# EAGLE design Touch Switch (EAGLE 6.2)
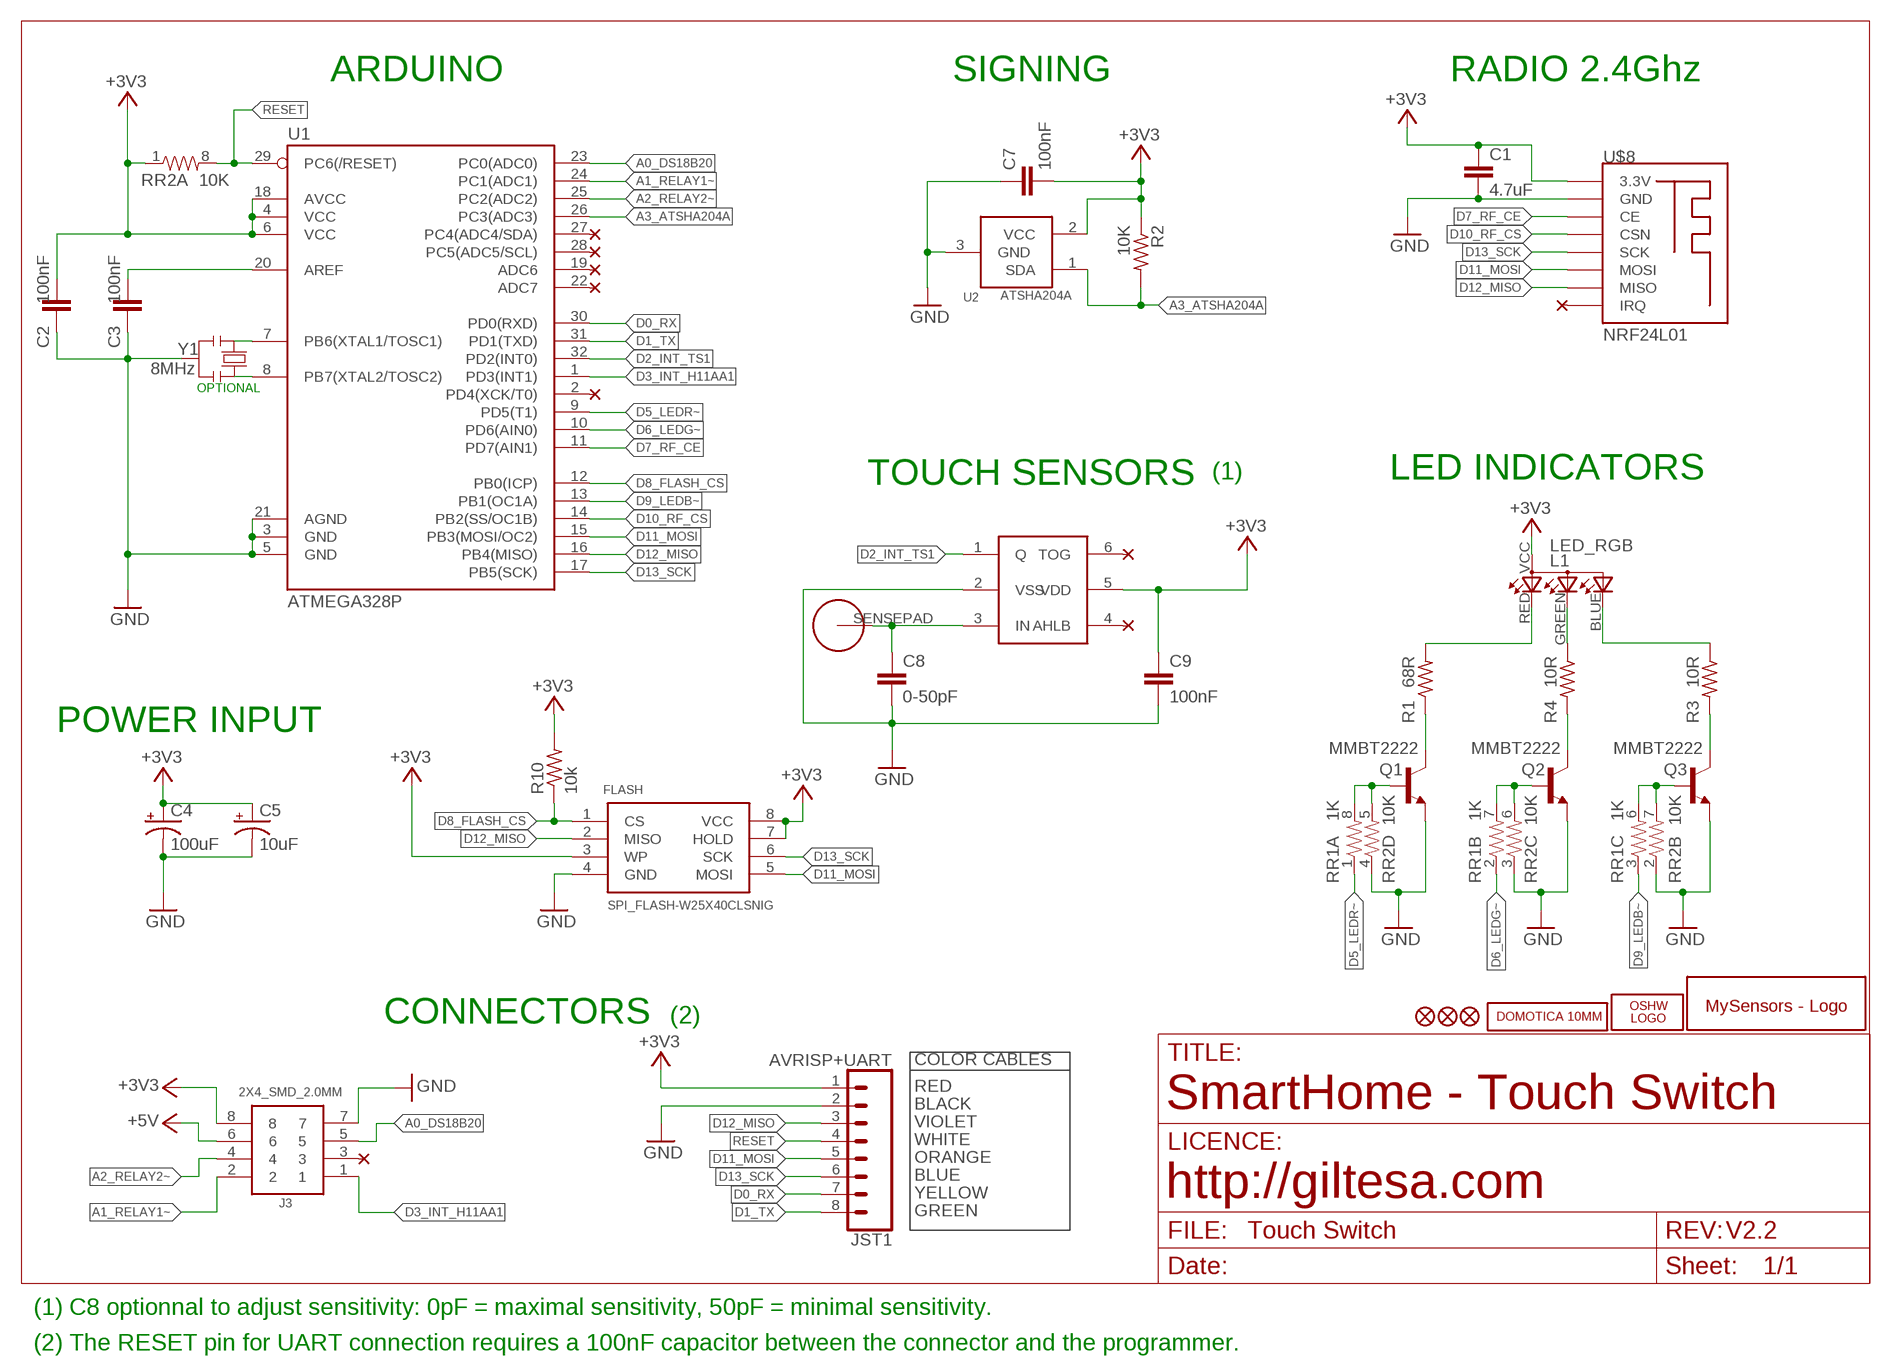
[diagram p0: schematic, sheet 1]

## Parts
C1  4.7uF  C1206  [C1206]
C2  100nF  C0603  [C0603]
C3  100nF  C0603  [C0603]
C4  100uF  10UF-16V-10%(TANT)  [EIA3216]
C5  10uF  10UF-16V-10%(TANT)  [EIA3216]
C7  100nF  C0603  [C0603]
C8  0-50pF  C0603  [C0603]
C9  100nF  C0603  [C0603]
FLASH  SPI_FLASH-W25X40CLSNIG  SPI_FLASH-X25XXSMD  [SO08]
J3  2X4_SMD_2.0MM  [2X4_SMD_2.0MM]
JST1  AVRISP+UART  JST-8-1MM-SMD  [JST-8-1MM-SMD]
L1  LED_RGB  LED_RGB_1206_SIDE  [LED_RGB_1206_SIDE]
LOGO1  OSHW_LOGO_FILLX0150-NT  [OSHW_FILLX150_NOTEXT]
Q1  MMBT2222  TRANSISTOR_NPNSOT23  [SOT23]
Q2  MMBT2222  TRANSISTOR_NPNSOT23  [SOT23]
Q3  MMBT2222  TRANSISTOR_NPNSOT23  [SOT23]
R1  68R  R0603  [R0603]
R2  10K  R0603  [R0603]
R3  10R  R0603  [R0603]
R4  10R  R0603  [R0603]
R10  10k  R0603  [R0603]
RR1  1K  RESISTOR-ARRAY0603-ARV  [0603-ARV]
RR2  10K  RESISTOR-ARRAY0603-ARV  [0603-ARV]
TTP1  TTP223  TTP223-BA6  [SOT-23-6]
U1  ATMEGA328P  ATMEGA328P_TQFP  [TQFP32-08]
U2  ATSHA204A  IC_ATSHA204A_CRYPT  [SOT23-3]
U$1  HTTM_SENSEPAD  [HTTM_SENSEPAD]
U$2  MYSENSORS  [MYSENSORS]
U$5  DOMOTICA-10MM  [DOMOTICA-10MM]
U$6  FIDUCIAL1X2  [FIDUCIAL-1X2]
U$7  FIDUCIAL1X2  [FIDUCIAL-1X2]
U$8  NRF24L01  NRF24L01_SMD  [NRF24L01_SMD]
U$14  FIDUCIAL1X2  [FIDUCIAL-1X2]
Y1  8MHz  RESONATORMU  [RESONATOR]

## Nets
+3V3: C1.1 C2.2 C4.A(+) C5.A(+) C7.2 C9.1 FLASH.3(WP) FLASH.7(HOLD) FLASH.8(VCC) J3.8 JST1.1 L1.VCC R2.1 R10.2 RR2.1 TTP1.5(VDD) U1.4(VCC) U1.6(VCC) U1.18(AVCC) U2.2(VCC) U$8.3.3V
+5V: J3.6
A0_DS18B20: J3.5 U1.23(PC0(ADC0))
A1_RELAY1~: J3.2 U1.24(PC1(ADC1))
A2_RELAY2~: J3.4 U1.25(PC2(ADC2))
A3_ATSHA204A: R2.2 U1.26(PC3(ADC3)) U2.1(SDA)
D0_RX: JST1.7 U1.30(PD0(RXD))
D1_TX: JST1.8 U1.31(PD1(TXD))
D2_INT_TS1: TTP1.1(Q) U1.32(PD2(INT0))
D3_INT_H11AA1: J3.1 U1.1(PD3(INT1))
D5_LEDR~: RR1.1 U1.9(PD5(T1))
D6_LEDG~: RR1.2 U1.10(PD6(AIN0))
D7_RF_CE: U1.11(PD7(AIN1)) U$8.CE
D8_FLASH_CS: FLASH.1(CS) R10.1 U1.12(PB0(ICP))
D9_LEDB~: RR1.3 U1.13(PB1(OC1A))
D10_RF_CS: U1.14(PB2(SS/OC1B)) U$8.CSN
D11_MOSI: FLASH.5(MOSI) JST1.5 U1.15(PB3(MOSI/OC2)) U$8.MOSI
D12_MISO: FLASH.2(MISO) JST1.3 U1.16(PB4(MISO)) U$8.MISO
D13_SCK: FLASH.6(SCK) JST1.6 U1.17(PB5(SCK)) U$8.SCK
GND: C1.2 C2.1 C3.1 C4.C(-) C5.C(-) C7.1 C8.2 C9.2 FLASH.4(GND) J3.7 JST1.2 Q1.2(E) Q2.2(E) Q3.2(E) RR2.2 RR2.3 RR2.4 TTP1.2(VSS) U1.3(GND) U1.5(GND) U1.21(AGND) U2.3(GND) U$8.GND Y1.2
N$1: Q1.3(C) R1.1
N$2: L1.GREEN R4.1
N$4: L1.RED R1.2
N$5: Q2.1(B) RR1.7 RR2.6
N$6: Q1.1(B) RR1.8 RR2.5
N$7: Q2.3(C) R4.2
N$8: Q3.3(C) R3.2
N$9: Q3.1(B) RR1.6 RR2.7
N$10: C8.1 TTP1.3(IN) U$1.SENSEPAD
N$11: L1.BLUE R3.1
N$29: U1.7(PB6(XTAL1/TOSC1)) Y1.1
N$30: U1.8(PB7(XTAL2/TOSC2)) Y1.3
N$33: C3.2 U1.20(AREF)
RESET: JST1.4 RR2.8 U1.29(PC6(/RESET))
Unconnected: J3.3 RR1.4 RR1.5 TTP1.4(AHLB) TTP1.6(TOG) U1.2(PD4(XCK/T0)) U1.19(ADC6) U1.22(ADC7) U1.27(PC4(ADC4/SDA)) U1.28(PC5(ADC5/SCL)) U$8.IRQ

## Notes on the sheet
- ARDUINO | SIGNING | RADIO 2.4Ghz
- OPTIONAL
- TOUCH SENSORS | (1) | LED INDICATORS
- POWER INPUT
- CONNECTORS | (2)
- COLOR CABLES
- RED
- BLACK | SmartHome - Touch Switch
- VIOLET
- WHITE
- ORANGE
- BLUE
- YELLOW | http://giltesa.com
- GREEN
- V2.2
- (1) C8 optionnal to adjust sensitivity: 0pF = maximal sensitivity, 50pF = minimal sensitivity.
- (2) The RESET pin for UART connection requires a 100nF capacitor between the connector and the programmer.

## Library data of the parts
C1 = ,giltesa:C1206
C2 C3 C7-C9 = ,giltesa:C0603
C4 = SparkFun-Capacitors:10UF-16V-10%(TANT): CAP-00811; PROD_ID: CAP-00811; VALUE: 10uF
C5 = SparkFun-Capacitors:10UF-16V-10%(TANT): CAP-00811; PROD_ID: CAP-00811
FLASH = SparkFun-DigitalIC:SPI_FLASH-X25XX: 8pin SPI Flash series x25xx. Works with devices like W25X32 and BR25L32
J3 = ,giltesa:2X4_SMD_2.0MM
JST1 = ,giltesa:JST-8-1MM-SMD
L1 = ,giltesa:LED_RGB_1206_SIDE
LOGO1 = ohw-logo:OSHW_LOGO_FILL
Q1-Q3 = SparkFun:TRANSISTOR_NPN: Transistor NPN BJT configuration in SOT23 package. MMBT2222 is the common NPN we use. Double check BCE configuration again layout.
R1-R4 R10 = ,giltesa:R0603
RR1 RR2 = SparkFun-Passives:RESISTOR-ARRAY: Array Chip Resistor Source: RS Component / Phycomp
TTP1 = NCA_Sensors:TTP223-BA6: TTP223 touch sensor
U1 = SparkFun-DigitalIC:ATMEGA328P_TQFP; PROD_ID: IC-09069; VALUE: ATMEGA328P_TQFP
U2 = TD-MySensors:IC_ATSHA204A_CRYPT
U$1 = ,giltesa:HTTM_SENSEPAD
U$2 = ,giltesa_logos:MYSENSORS
U$5 = ,giltesa_logos:DOMOTICA-10MM
U$6 U$7 U$14 = SparkFun:FIDUCIAL: Fiducial Alignment Points
U$8 = ,giltesa:NRF24L01_SMD
Y1 = MySMD2:RESONATOR

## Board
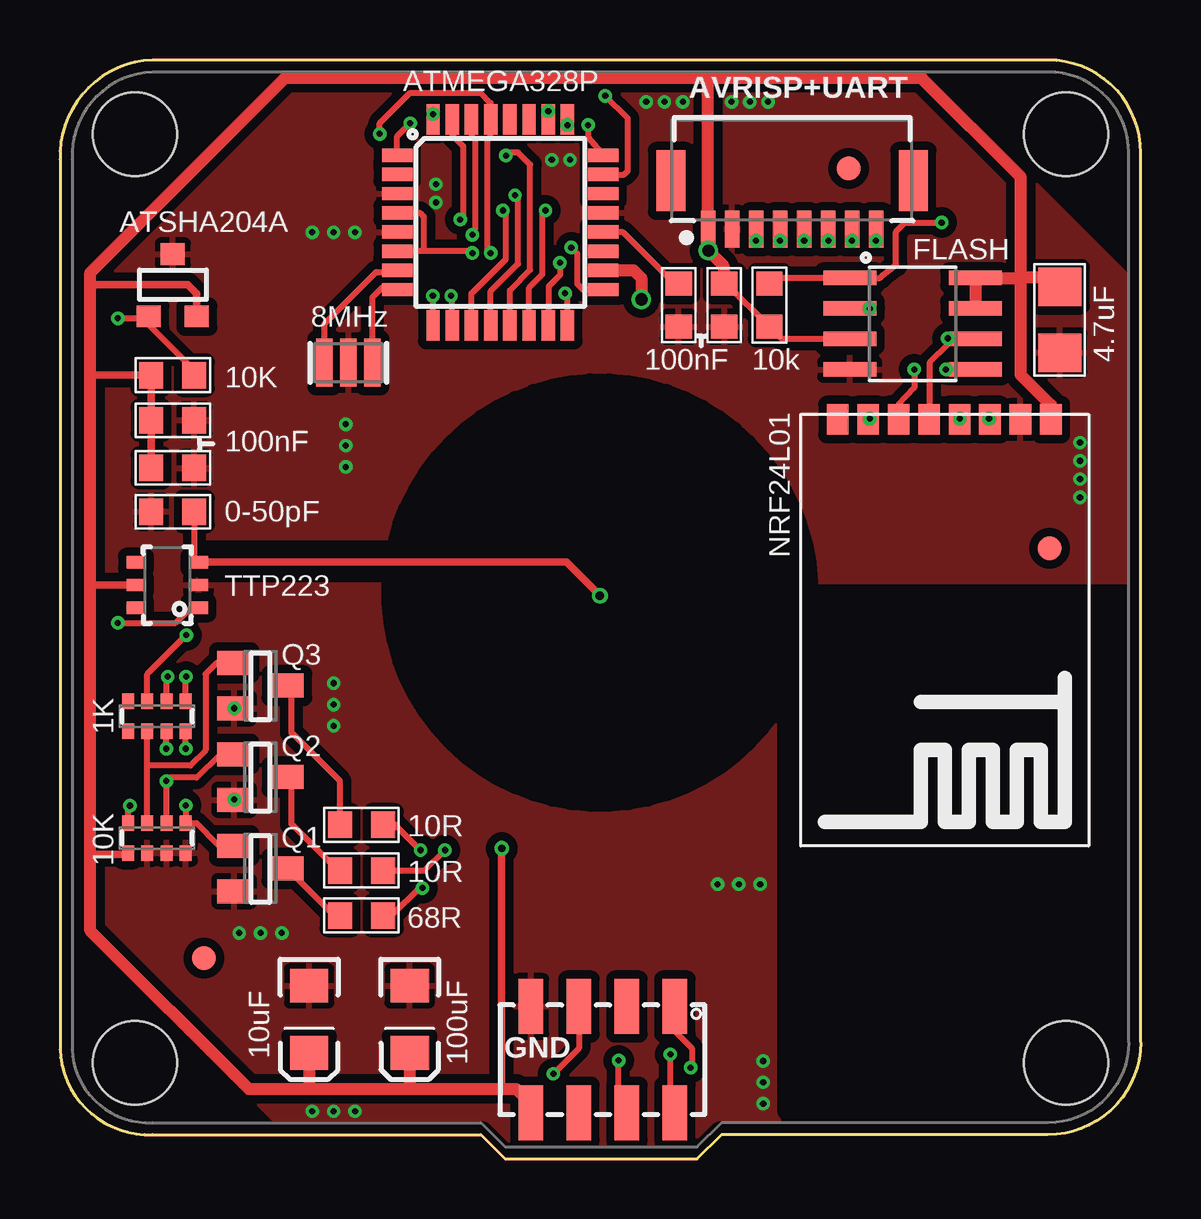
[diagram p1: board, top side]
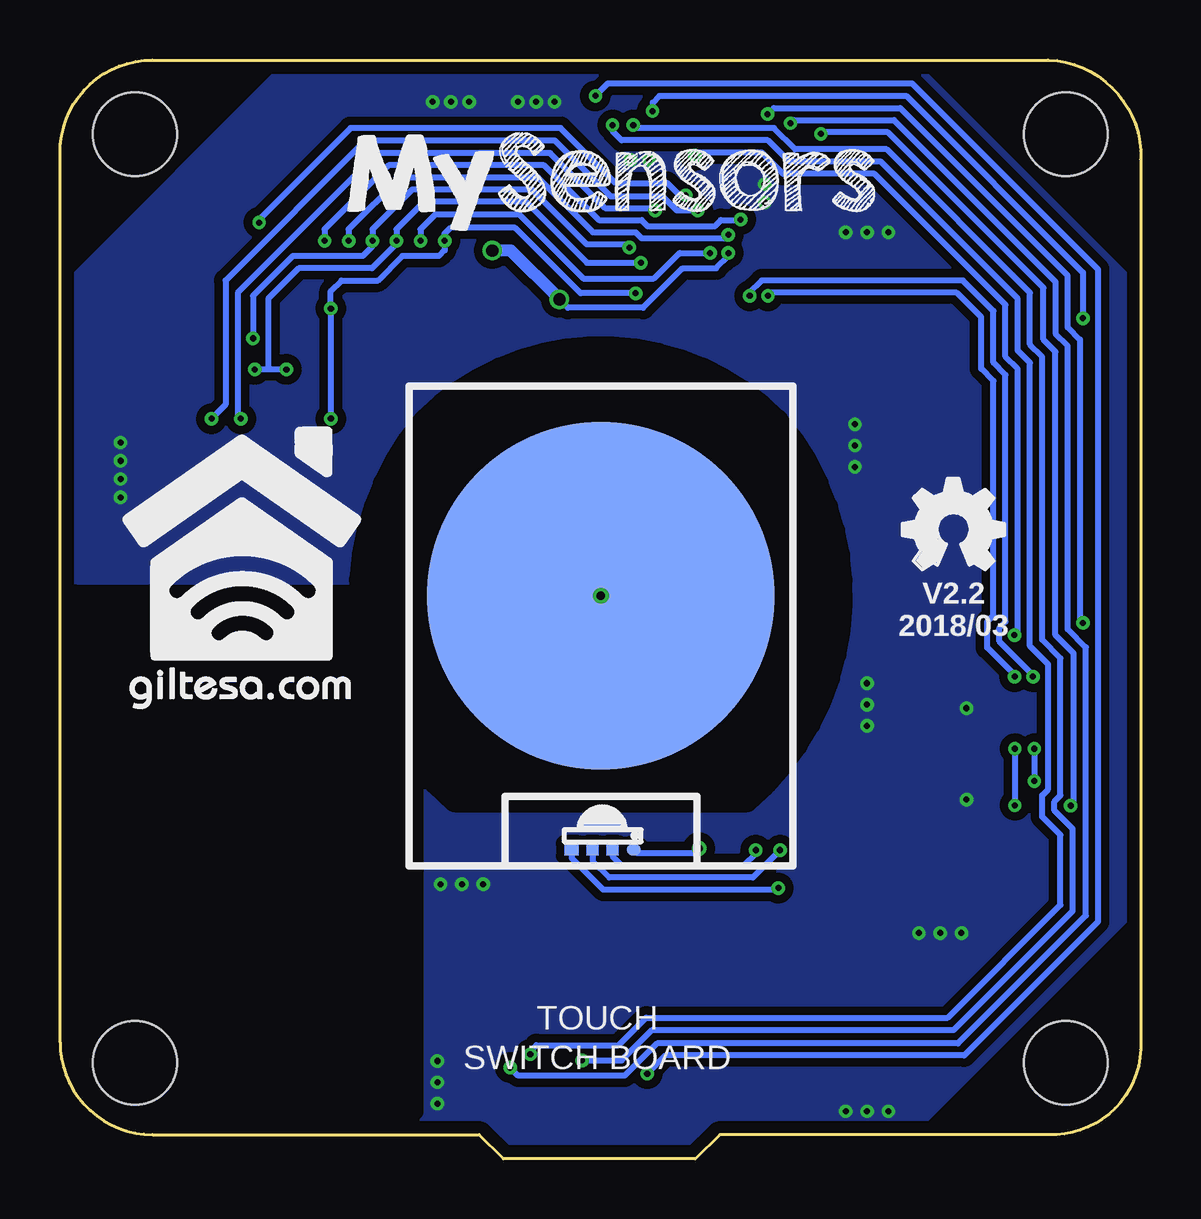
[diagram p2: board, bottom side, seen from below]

Size 45.05 x 45.81 mm. Coordinates in mm from the lower left corner, seen from the top.
Outline: 18.56,0 26.56,0 27.58,1.02 41.19,1.02 arc90 45.05,4.87 45.05,41.96 arc90 41.19,45.81 3.86,45.81 arc90 0,41.66 0,4.57 arc90 3.86,1.02 17.55,1.02 18.56,0
Copper layers (1*16): Top 0.035mm / dielectric 1.6mm / Bottom 0.035mm
Design rules: minimum track width 6mil, minimum drill 12mil, track to track 6mil, track to pad 6mil, pad to pad 6mil, via to via 8mil, smd to smd 0mil, copper to edge 20mil, drill to drill 10mil, minimum pad ring 6mil, minimum via ring 6mil, stop-mask expansion 0mil, vias tented up to drill 100mil, thermal gap 10mil
Holes 3.5 mm at 3.12,4.01 41.93,42.72 3.12,42.72 41.93,4.01
tRestrict: area 13.9,14.9 to 31.1,32.3; area 6.1,24.4 to 13.8,25.4; area 30.3,2 to 44.4,23.5
bRestrict: area 12.5,14.9 to 32.6,33.8; area 30.3,2 to 44.4,23.5

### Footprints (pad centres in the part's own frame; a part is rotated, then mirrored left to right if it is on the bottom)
C1206 = smd 1.6 x 1.8: 1 -1.362,-0.013; 2 1.387,-0.013
C0603 = smd 1 x 1.1: 1 -0.901,-0.038; 2 0.901,-0.038
EIA3216 = smd 1.4 x 1.6: A 1.4,0; C -1.4,0
SO08 = smd 0.61 x 2.21: 1 -1.905,-2.616; 2 -0.635,-2.616; 3 0.635,-2.616; 4 1.905,-2.616; 5 1.905,2.616; 6 0.635,2.616; 7 -0.635,2.616; 8 -1.905,2.616
2X4_SMD_2.0MM = smd 2.286 x 1.016: 1 -2.213,2.976; 2 2.212,2.976; 3 -2.213,0.976; 4 2.212,0.976; 5 -2.213,-1.024; 6 2.212,-1.024; 7 -2.213,-3.024; 8 2.212,-3.024
JST-8-1MM-SMD = smd 0.6 x 1.55: 1 -3.5,-2.017; 2 -2.5,-2.017; 3 -1.5,-2.017; 4 -0.5,-2.017; 5 0.5,-2.017; 6 1.5,-2.017; 7 2.5,-2.017; 8 3.5,-2.017 | smd 1.219 x 2.54: P$9 5.054,0; P$10 -5.054,0
LED_RGB_1206_SIDE = smd 0.5 x 0.5: BLUE -0.419,-0.83; GREEN 0.414,-0.83 | smd 0.6 x 0.5: RED -1.296,-0.83; VCC 1.295,-0.83
SOT23 = smd 1 x 1.4: 1 -0.95,-1.1; 2 0.95,-1.1; 3 0,1.1
R0603 = smd 1 x 1.1: 1 -0.901,0.013; 2 0.901,0.013
0603-ARV = smd 0.5 x 0.65: 1 -1.2,-0.625; 2 -0.4,-0.625; 3 0.4,-0.625; 4 1.2,-0.625; 5 1.2,0.625; 6 0.4,0.625; 7 -0.4,0.625; 8 -1.2,0.625
SOT-23-6 = smd 0.51 x 0.8: 1 0.955,-0.03; 2 1.905,-0.03; 3 2.855,-0.03; 4 2.855,2.57; 5 1.905,2.57; 6 0.955,2.57
TQFP32-08 = smd 1.27 x 0.559: 1 -4.293,2.8; 2 -4.293,2; 3 -4.293,1.2; 4 -4.293,0.4; 5 -4.293,-0.4; 6 -4.293,-1.2; 7 -4.293,-2; 8 -4.293,-2.8; 17 4.293,-2.8; 18 4.293,-2; 19 4.293,-1.2; 20 4.293,-0.4; 21 4.293,0.4; 22 4.293,1.2; 23 4.293,2; 24 4.293,2.8 | smd 0.559 x 1.27: 9 -2.8,-4.293; 10 -2,-4.293; 11 -1.2,-4.293; 12 -0.4,-4.293; 13 0.4,-4.293; 14 1.2,-4.293; 15 2,-4.293; 16 2.8,-4.293; 25 2.8,4.293; 26 2,4.293; 27 1.2,4.293; 28 0.4,4.293; 29 -0.4,4.293; 30 -1.2,4.293; 31 -2,4.293; 32 -2.8,4.293
SOT23-3 = smd 1 x 0.9: 1 -1,-1.3; 2 1,-1.3; 3 0,1.3
HTTM_SENSEPAD = smd 14.5 x 14.5: SENSEPAD -0.001,0.001
FIDUCIAL-1X2 = smd 1 x 1: 1 0,0
NRF24L01_SMD = smd 0.9 x 1.27: 3.3V 1.575,0.203; CE 4.115,0.203; CSN 5.385,0.203; GND 2.845,0.203; IRQ 10.465,0.203; MISO 9.195,0.203; MOSI 7.925,0.203; SCK 6.655,0.203
RESONATOR = smd 0.7 x 2: 1 -1,0; 2 0,0; 3 1,0

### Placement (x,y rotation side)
C1  41.69,35 270 top
C2  27.65,35.59 90 top
C3  25.75,35.59 90 top
C4  14.58,5.83 270 top
C5  10.38,5.83 270 top
C7  4.7,30.75 180 top
C8  4.7,26.94 180 top
C9  4.7,28.85 0 top
FLASH  35.54,34.82 270 top
J3  22.66,4.15 270 top
JST1  30.52,40.77 0 top
L1  22.43,13.73 0 bottom
LOGO1  9.93,24.56 0 bottom
Q1  8.36,12.11 270 top
Q2  8.36,15.92 270 top
Q3  8.36,19.73 270 top
R1  12.57,10.14 0 top
R2  4.7,32.66 0 top
R3  12.57,13.95 180 top
R4  12.57,12.04 180 top
R10  29.56,35.59 270 top
RR1  4.04,18.46 180 top
RR2  4.04,13.38 0 top
TTP1  5.74,22.02 90 top
U1  18.35,39.04 0 top
U2  4.7,36.42 0 top
U$1  22.5,23.48 0 bottom
U$2  33.05,38.5 0 bottom
U$5  42.46,18.69 0 bottom
U$6  41.25,25.45 0 top
U$7  32.87,41.3 0 top
U$8  42.88,31.03 180 top
U$14  6,8.38 0 top
Y1  12.02,33.19 0 top

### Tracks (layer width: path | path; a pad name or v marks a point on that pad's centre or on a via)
+3V3  (via drill 0.25, 0.3, 0.51)
  Top 0.254: U1.6 14.09,37.87 15.16,37.87 | U1.4 15.01,39.44 15.16,39.29 15.16,37.87 | C2.2 27.77,36.49 R10.2 | 29.95,34.31 R10.2 | FLASH.3 30.08,34.18 R10.2 | 15.16,37.87 17.09,37.87 v17.19,37.77
  Top 0.305: RR2.1 2.78,12.7 1.27,12.7 | TTP1.5 1.34,23.93 1.27,24 | C9.1 C7.2 R2.1 1.35,32.67 1.27,32.76 | U2.2 5.7,36.07 5.33,36.44 1.39,36.44 1.27,36.32 | v18.41,12.95 18.41,2.99 18.33,2.92
  Top 0.508: C2.2 27.65,37.24 v27.03,37.87 | 29.77,34.74 R10.2 | 26.84,45.08 9.39,45.08 1.27,36.95 1.27,36.32 1.27,32.76 1.27,24 1.27,12.7 1.27,9.52 7.87,2.92 10.33,2.92 | 26.84,45.08 35.91,45.08 40.05,40.94 40.05,36.88 | 10.33,2.92 14.52,2.92 | 14.52,2.92 18.33,2.92 19.02,2.92 19.48,2.46 19.48,2.09 J3.8 | C5.A 10.38,2.97 10.33,2.92 | C4.A 14.58,2.97 14.52,2.92 | 26.84,45.08 27.02,45.03 JST1.1 27.02,38.51 v27.03,37.87 | U$8.3.3V 41.3,31.43 40.05,32.69 40.05,36.62 | 41.68,36.34 C1.1 41.57,36.26 41.57,36.24 41.07,36.75 40.18,36.75 40.05,36.88 | FLASH.7 FLASH.8 39.95,36.72 40.05,36.62 | 40.05,36.62 40.05,36.88 | v24.23,35.84 24.23,36.72 23.92,37.04 U1.18 | 27.02,38.64 v27.03,37.87
  Bottom 0.254: v18.41,12.95 18.39,12.95 18.59,12.75 20.98,12.75 L1.VCC | v24.23,35.84 23.88,35.48 20.75,35.48 19.1,37.13 17.7,37.13 17.19,37.64 v17.19,37.77
  Bottom 0.508: v24.23,35.84 26.27,37.87 v27.03,37.87
A0_DS18B20  (via drill 0.25)
  Top 0.254: 21.46,7.08 J3.5 21.63,4.61 v20.57,3.55 | U1.23 23.51,41.04 23.67,41.19 23.67,43.38 v22.73,44.32
  Bottom 0.254: v22.73,44.32 22.22,44.83 9.52,44.83 1.77,37.08 1.77,9.9 7.36,4.31 19.81,4.31 v20.57,3.55
A1_RELAY1~  (via drill 0.25)
  Top 0.254: J3.2 25.63,2.15 25.45,2.33 v25.45,4.36 | 22.64,41.83 U1.24 22.02,42.6 v22.02,43.1
  Bottom 0.254: v25.45,4.36 25.45,4.49 25.19,4.75 21.76,4.75 20.62,5.89 8.05,5.89 3.35,10.59 3.35,13.51 4.11,14.27 4.11,15.16 3.86,15.41 3.86,20.62 4.62,21.38 4.62,33.19 5.13,33.7 5.13,35.86 10.84,41.58 14.65,41.58 15.54,42.46 21.64,42.46 22.02,42.84 v22.02,43.1
A2_RELAY2~  (via drill 0.25)
  Top 0.254: J3.4 23.63,1.99 23.29,2.33 v23.29,4.11 | v21.15,43.1 21.13,43.31 U1.25
  Bottom 0.254: v23.29,4.11 21.64,4.11 20.37,5.38 7.79,5.38 2.84,10.33 2.84,13.76 3.6,14.52 3.6,14.9 3.35,15.16 3.35,20.87 4.11,21.64 4.11,33.45 4.62,33.95 4.62,36.11 10.59,42.08 14.4,42.08 15.29,42.97 21,42.97 v21.15,43.1
A3_ATSHA204A  (via drill 0.25)
  Top 0.254: R2.2 5.31,32.9 5.31,33.17 3.7,34.78 U2.1 3.63,35.05 v2.41,35.05 | U1.26 20.35,43.65 v20.35,43.68
  Bottom 0.254: v20.35,43.68 20.34,44.04 20.06,44.32 9.78,44.32 2.41,36.95 v2.41,35.05
D0_RX  (via drill 0.25)
  Top 0.254: U1.30 17.15,42.63 17.32,42.46 17.32,38.78 17.19,38.65 v17.19,38.53 | v33.02,38.27 33.07,38.71 JST1.7
  Bottom 0.254: v33.02,38.27 33.02,38.32 JST1.7 30.86,40.91 25.12,40.91 22.84,38.63 21.06,38.63 20.8,38.38 17.34,38.38 v17.19,38.53
D1_TX  (via drill 0.25)
  Top 0.254: v34.02,38.27 34.01,38.69 JST1.8 | U1.31 16.35,42.67 16.81,42.21 16.81,39.29 v16.68,39.16
  Bottom 0.254: v34.02,38.27 34.02,38.34 JST1.8 31.35,41.42 24.87,41.42 22.58,39.14 20.8,39.14 20.55,38.88 17.76,38.88 17.5,39.14 16.84,39.14 v16.68,39.16
D2_INT_TS1  (via drill 0.25)
  Top 0.254: U1.32 15.55,43.37 v15.55,43.56 | v2.41,22.35 4.82,22.35 5.45,22.98 TTP1.1
  Bottom 0.254: v15.55,43.56 15.3,43.81 10.03,43.81 3.04,36.83 3.04,34.67 2.54,34.16 2.54,22.47 v2.41,22.35
D3_INT_H11AA1  (via drill 0.25)
  Top 0.254: U1.1 14.06,42.63 v14.6,43.17 | J3.1 25.52,7.15 25.52,5.43 26.34,4.62 26.34,3.86 v26.29,3.81
  Bottom 0.254: v14.6,43.17 14.47,43.3 10.28,43.3 3.55,36.57 3.55,34.41 3.04,33.9 3.04,22.09 2.28,21.33 2.28,10.15 7.62,4.82 20.16,4.82 21.51,3.48 25.95,3.48 v26.29,3.81
D5_LEDR~  (via drill 0.25)
  Top 0.254: RR1.1 v5.24,20.1 v5.25,20.11 | v15.54,35.99 15.54,34.76 U1.9
  Bottom 0.254: v5.25,20.11 5.25,20.18 6.4,21.32 6.4,22.4 6.14,22.65 6.14,32.43 6.65,32.94 6.65,35.1 7.67,36.11 15.41,36.11 v15.54,35.99
D6_LEDG~  (via drill 0.25)
  Top 0.254: RR1.2 4.44,20.06 v4.49,20.11 | U1.10 16.35,35.94 v16.3,35.99
  Bottom 0.254: v4.49,20.11 4.49,20.18 5.89,21.57 5.89,22.14 5.63,22.4 5.63,32.69 6.14,33.19 6.14,35.35 7.41,36.62 15.79,36.62 16.3,36.11 v16.3,35.99
D7_RF_CE  (via drill 0.25)
  Top 0.254: v38.73,30.86 U$8.CE | U1.11 17.15,36.08 18.59,37.51 18.59,39.42 v18.46,39.54
  Bottom 0.254: v38.73,30.86 38.15,31.44 38.15,36.62 32.3,42.46 24.43,42.46 22.09,40.13 19.93,40.13 19.35,39.54 v18.46,39.54
D8_FLASH_CS  (via drill 0.25)
  Top 0.254: v36.75,39.03 35.22,39.03 34.84,38.65 34.84,37.26 34.31,36.85 34.18,36.72 FLASH.1 29.8,36.72 R10.1 | U1.12 17.95,36.18 19.1,37.32 19.1,40.05 v18.97,40.18
  Bottom 0.254: v36.75,39.03 36.75,39.16 32.94,42.97 24.18,42.97 21.89,40.69 19.73,40.69 19.22,40.18 v18.97,40.18
D9_LEDB~  (via drill 0.25)
  Top 0.254: U1.13 18.75,36.22 19.6,37.07 19.6,41.45 19.1,41.96 18.71,41.96 v18.59,41.83 | RR1.3 3.64,20.21 v5.27,21.84
  Bottom 0.254: v5.27,21.84 5.18,21.84 5.13,21.89 5.13,32.94 5.63,33.45 5.63,35.61 11.1,41.07 14.91,41.07 15.79,41.96 18.46,41.96 v18.59,41.83
D10_RF_CS  (via drill 0.25)
  Top 0.254: v37.51,30.86 v37.51,30.85 U$8.CSN | U1.14 19.55,36.32 20.11,36.88 20.11,39.42 v20.24,39.54
  Bottom 0.254: v37.51,30.86 37.64,30.98 37.64,36.11 31.82,41.93 24.61,41.93 22.33,39.65 20.34,39.65 v20.24,39.54
D11_MOSI  (via drill 0.25)
  Top 0.254: FLASH.5 v36.93,32.91 | U$8.MOSI 34.95,31.44 35.61,32.15 v35.61,32.91 | v31.02,38.27 31.03,38.74 JST1.5 | v20.84,37.36 20.84,36.84 20.37,36.37 20.37,34.76 U1.15
  Bottom 0.254: 36.37,32.91 v35.61,32.91 35.61,32.79 | 36.37,32.91 v36.93,32.91 | 36.37,32.91 36.37,35.86 35.1,37.13 32.05,37.13 31.02,38.16 v31.02,38.27 31.02,38.29 JST1.5 29.88,39.9 25.63,39.9 23.09,37.36 v20.84,37.36
D12_MISO  (via drill 0.25)
  Top 0.254: U1.16 21.15,35.99 v21.06,36.09 | v33.76,35.45 FLASH.2 | v33.76,30.86 U$8.MISO | v29.02,38.27 29,38.74 JST1.3
  Bottom 0.254: v21.06,36.09 23.34,36.09 26.07,38.82 28.77,38.82 29.02,38.56 29.02,38.29 v29.02,38.27 29.02,37.88 29.26,37.64 30.78,37.64 31.8,36.62 33.32,36.62 33.76,36.18 v33.76,35.45 v33.76,30.86
D13_SCK  (via drill 0.25)
  Top 0.254: U1.17 21.8,36.24 21.57,36.47 21.57,37.74 v21.31,37.99 | v32.02,38.27 32.05,38.73 JST1.6 | U$8.SCK 36.27,30.85 36.27,33.22 37,33.95 v37,34.21 37.03,34.18 FLASH.6
  Bottom 0.254: v21.31,37.99 21.44,38.12 23.09,38.12 25.38,40.41 30.37,40.41 JST1.6 32.02,38.3 v32.02,38.27 32.02,38.04 32.43,37.64 35.35,37.64 37,35.99 v37,34.21
GND  (via drill 0.25)
  other vias: 42.52,29.87 42.52,29.1 42.52,28.34 42.52,27.58 7.27,18.79 7.27,14.98 27.99,44.06 28.75,44.06 29.52,44.06 25.96,44.06 25.2,44.06 24.44,44.06 15.67,40.64 29.19,11.45 28.3,11.45 27.41,11.45 29.31,2.31 29.31,3.2 29.31,4.08 7.47,9.42 8.36,9.42 9.25,9.42 11.41,19.83 11.41,18.94 11.41,18.05 10.52,1.99 11.41,1.99 12.3,1.99 11.91,30.63 11.91,29.74 11.91,28.85 10.52,38.63 11.41,38.63 12.3,38.63 20.5,41.65 21.26,41.65 15.67,39.87
  pour Bottom (isolate 0.356): 9.83,46.15 35.22,46.15 45.26,36.11 45.26,10.71 35.22,0.68 27.73,0.68 26.72,-0.33 18.33,-0.33 17.32,0.68 9.83,0.68 -0.21,10.71 -0.21,36.11
  pour Top (isolate 0.356): 9.83,46.15 35.22,46.15 45.26,36.11 45.26,10.71 35.22,0.68 27.73,0.68 26.72,-0.33 18.33,-0.33 17.32,0.68 9.83,0.68 -0.21,10.71 -0.21,36.11
N$1
  Top 0.254: R1.1 11.42,10.15 Q1.3
N$2  (via drill 0.25)
  Top 0.254: R4.1 15.2,12.03 v16.05,12.87
  Bottom 0.254: v16.05,12.87 16.05,12.75 16.56,12.24 21.64,12.24 22.02,12.62 L1.GREEN
N$4  (via drill 0.25)
  Top 0.254: R1.2 13.83,10.15 14.98,11.3 v15.11,11.3
  Bottom 0.254: v15.11,11.3 15.19,11.22 22.4,11.22 23.73,12.55 L1.RED
N$5  (via drill 0.25)
  Top 0.254: Q2.1 6.67,16.87 5.69,15.9 4.57,15.9 v4.43,15.76 RR2.6 4.48,14.05 | v4.43,17.1 RR1.7
  Bottom 0.254: v4.43,17.1 v4.43,15.76
N$6  (via drill 0.25)
  Top 0.254: Q1.1 6.62,13.06 5.69,13.99 5.13,13.99 RR2.5 5.25,13.89 v5.25,14.74 | v5.25,17.1 RR1.8
  Bottom 0.254: v5.25,17.1 v5.25,14.74
N$7
  Top 0.254: 11.58,12.03 9.65,13.96 9.65,15.73 Q2.3
  Top 0.406: R4.2 11.58,12.03
N$8
  Top 0.254: R3.2 11.67,15.76 9.65,17.77 9.65,19.54 Q3.3
N$9
  Top 0.254: RR2.7 3.64,16.4 | 3.64,16.4 RR1.6 | Q3.1 6.54,20.68 6.07,20.21 6.07,17.04 5.44,16.4 3.64,16.4
N$10  (via drill 0.36)
  Top 0.254: 5.55,24.88 TTP1.3 5.6,25.05 C8.1
  Top 0.305: TTP1.3 21.11,24.88 v22.5,23.48
  Bottom 0.127: U$1.SENSEPAD v22.5,23.48 | v22.5,23.48
  Bottom 0.305: v22.5,23.48 22.41,24.28
  Bottom 0.406: 22.46,24.18 v22.5,23.48
N$11  (via drill 0.25)
  Top 0.254: R3.1 13.97,13.93 v15.03,12.87
  Bottom 0.254: v15.03,12.87 16.18,11.73 22.14,11.73 22.85,12.44 L1.BLUE
N$29
  Top 0.254: Y1.1 11.02,34.81 13.18,36.98 14.14,36.98 | 14.14,36.98 14.45,36.98 | U1.7 14.12,37.1 14.12,36.99 14.14,36.98
N$30
  Top 0.254: Y1.3 13.02,35.93 13.44,36.34 13.96,36.34 U1.8
N$33
  Top 0.254: C3.2 25.66,36.44 23.47,38.63 U1.20
RESET  (via drill 0.25)
  Top 0.254: RR2.8 2.84,14.65 v2.92,14.73 | v13.33,42.73 13.33,43.17 14.6,44.45 17.52,44.45 17.95,44.01 U1.29 17.95,42.59 17.83,42.46 17.83,37.89 v17.95,37.77 | v30.02,38.27 JST1.4
  Bottom 0.254: v2.92,14.73 2.79,14.85 2.79,21.08 3.55,21.84 3.55,33.65 4.06,34.16 4.06,36.32 10.54,42.79 13.27,42.79 v13.33,42.73 | v30.02,38.27 JST1.4 29.41,39.37 25.9,39.37 23.24,36.7 20.29,36.7 19.22,37.77 v17.95,37.77

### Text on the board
tPlace: GND
bPlace: V2.2 | 2018/03 | TOUCH | SWITCH BOARD

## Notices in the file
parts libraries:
SparkFun-DigitalIC: Licensing: Creative Commons ShareAlike 4.0 International - https://creativecommons.org/licenses/by-sa/4.0
